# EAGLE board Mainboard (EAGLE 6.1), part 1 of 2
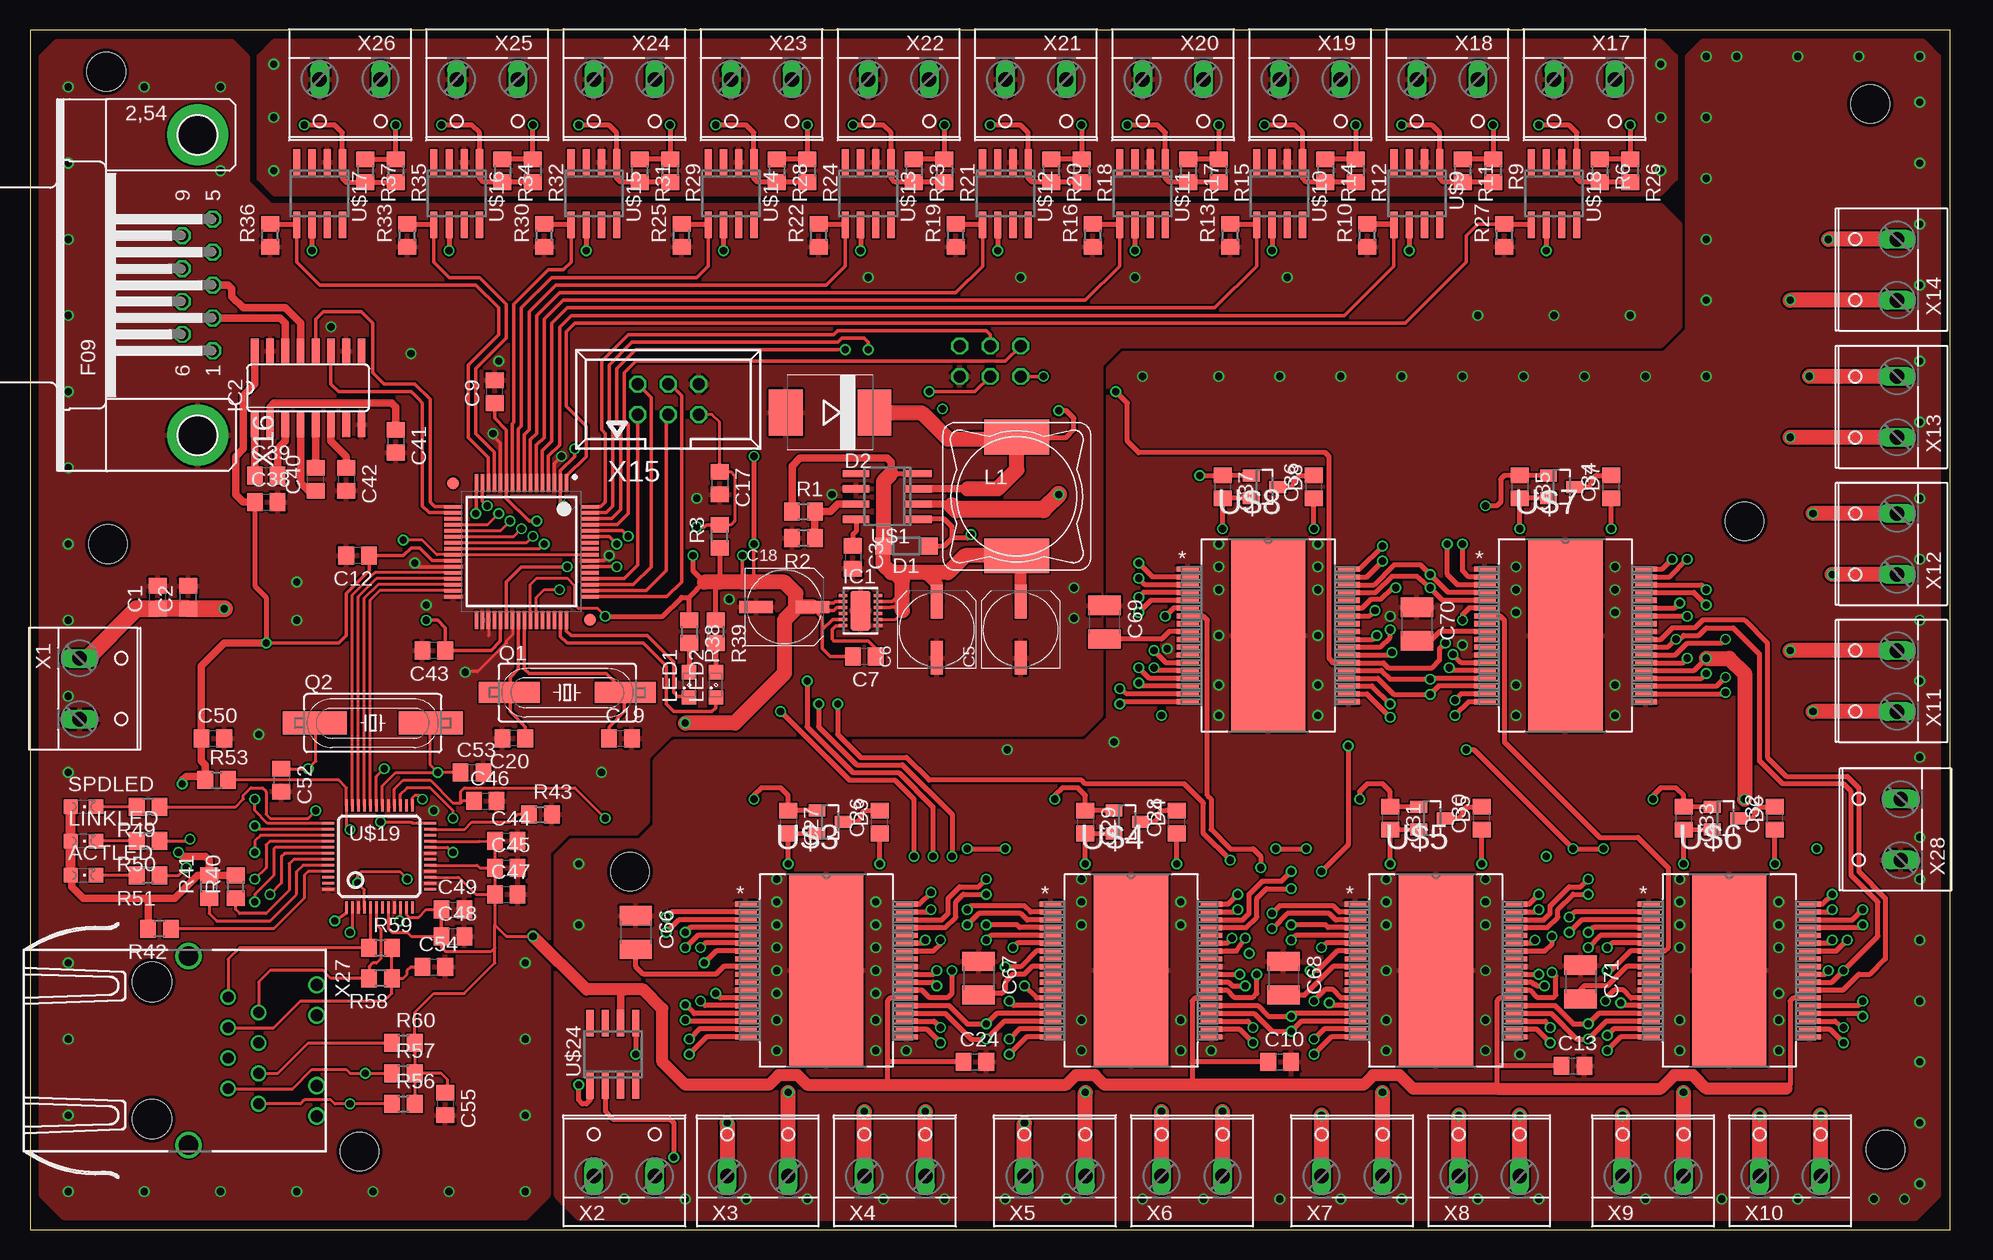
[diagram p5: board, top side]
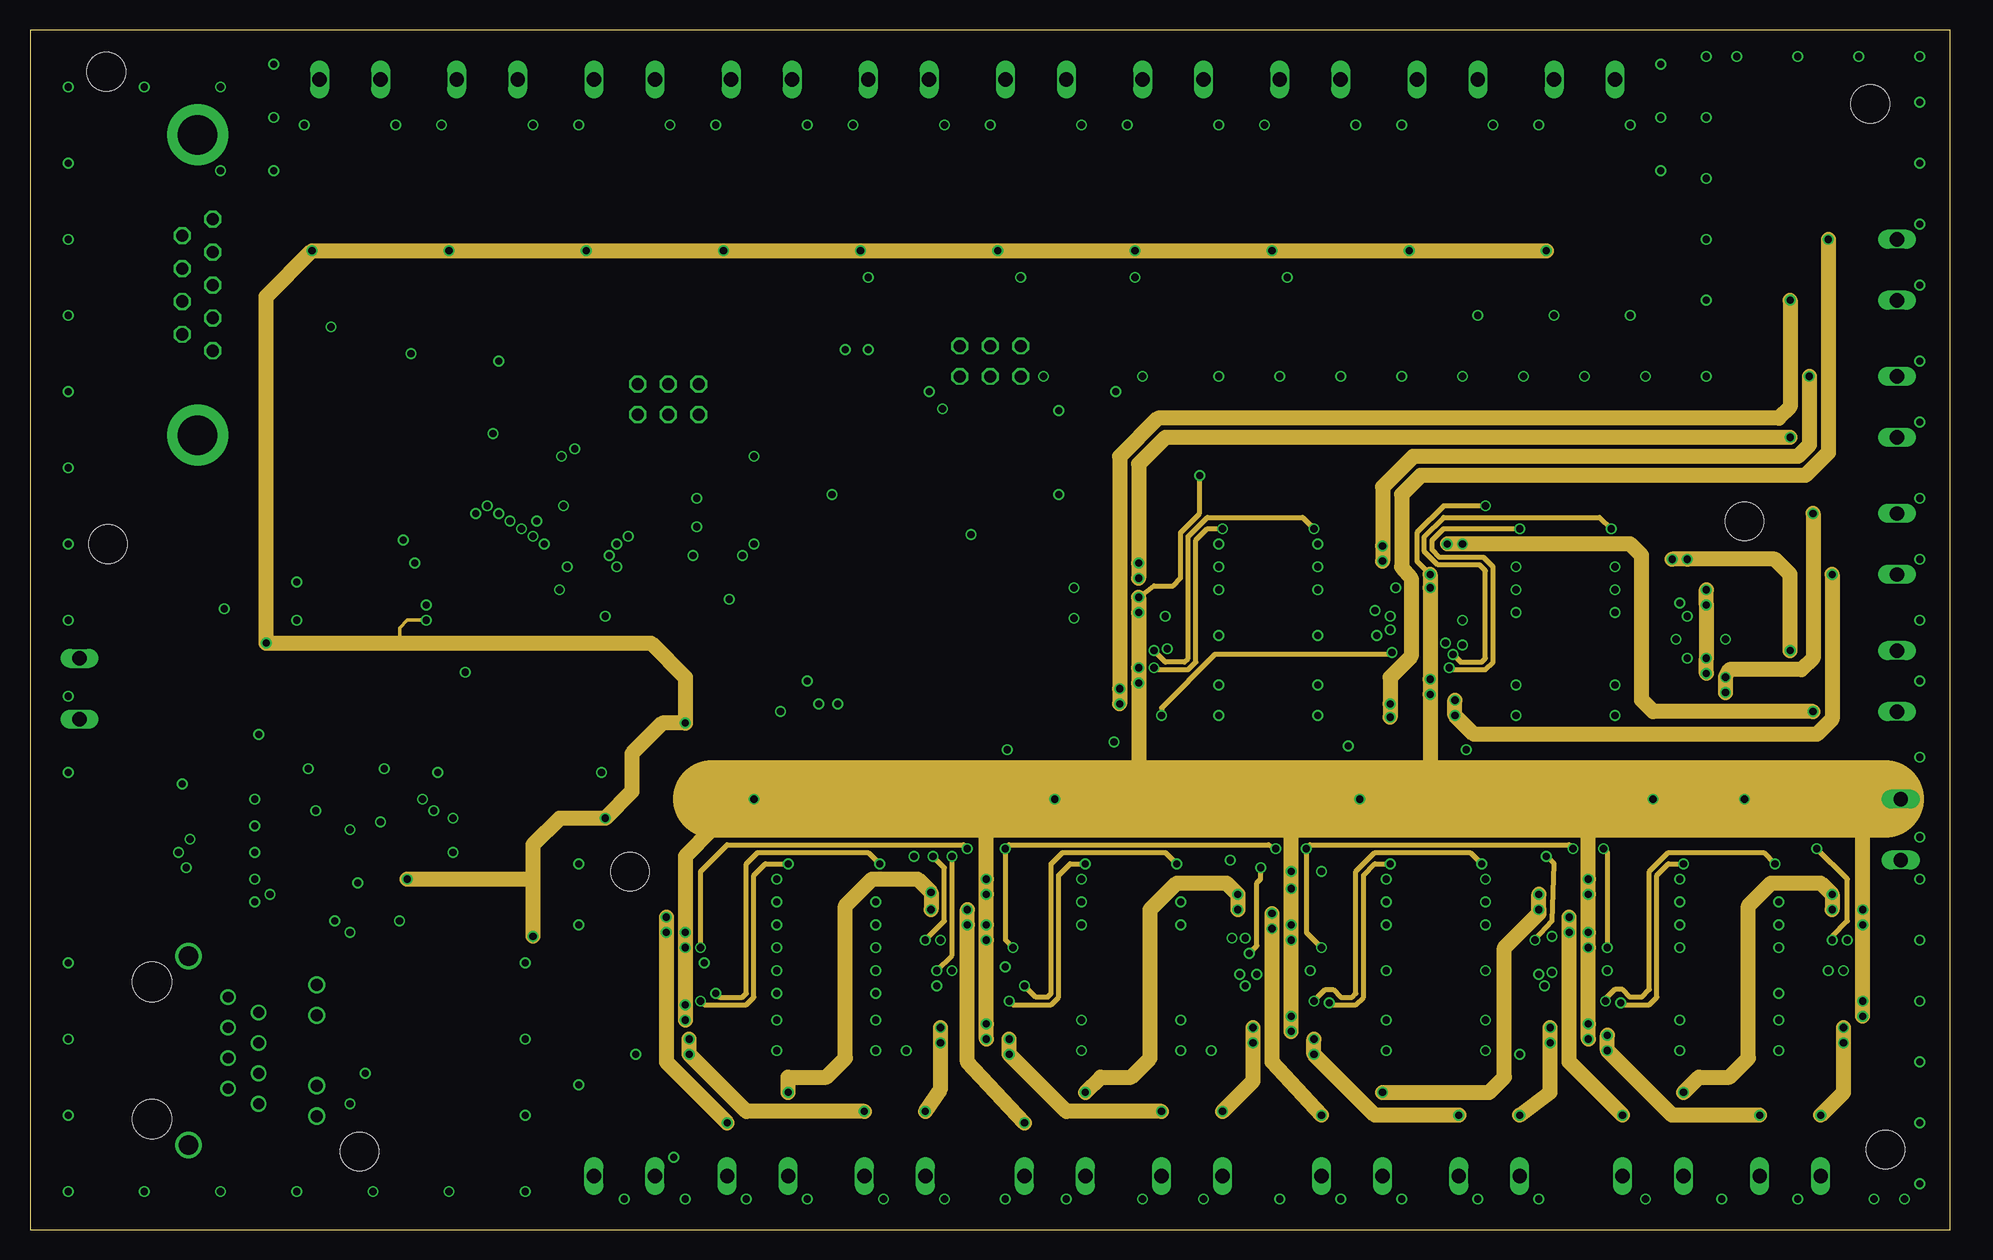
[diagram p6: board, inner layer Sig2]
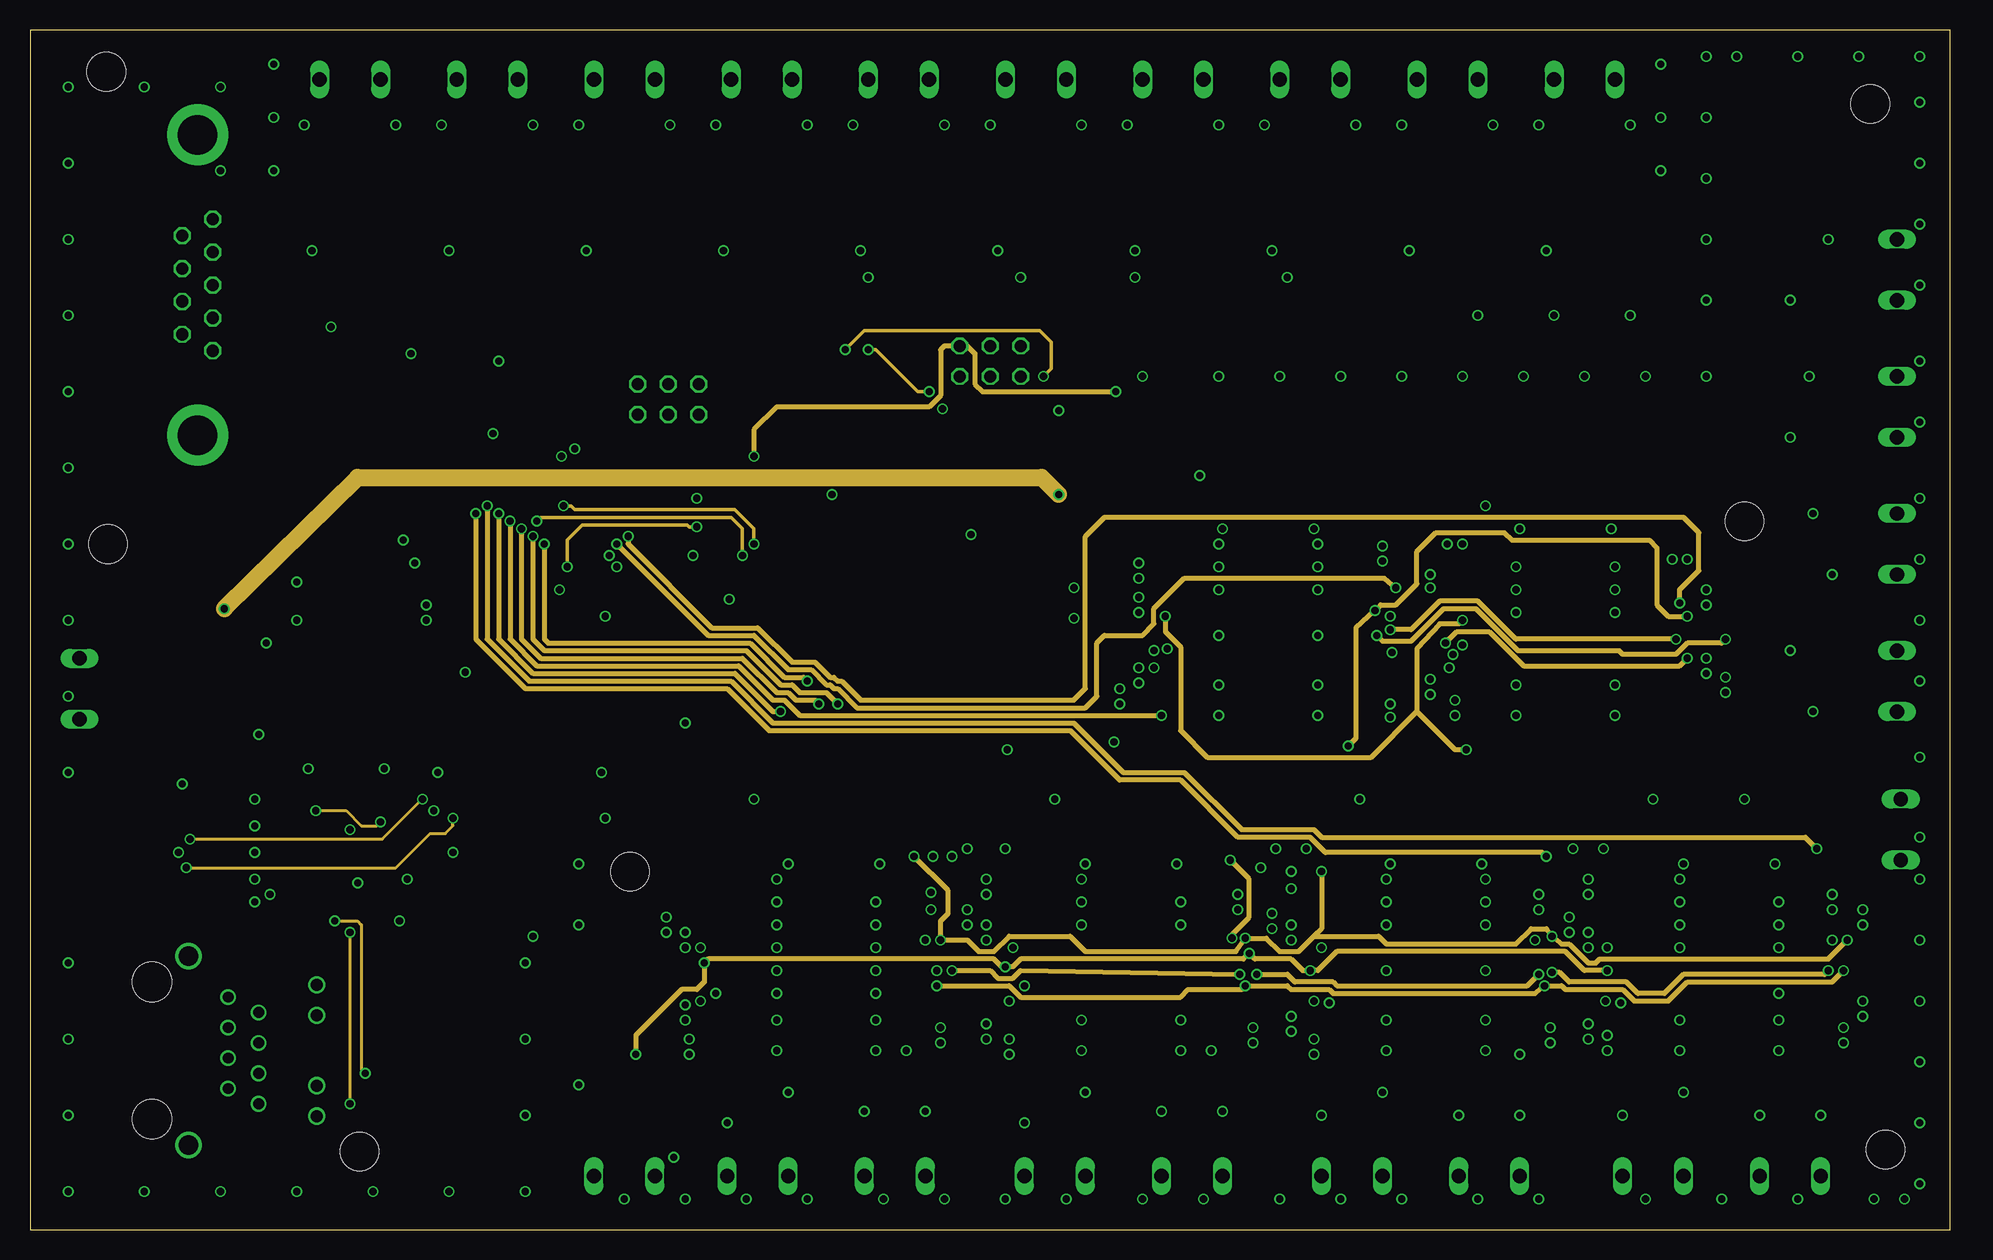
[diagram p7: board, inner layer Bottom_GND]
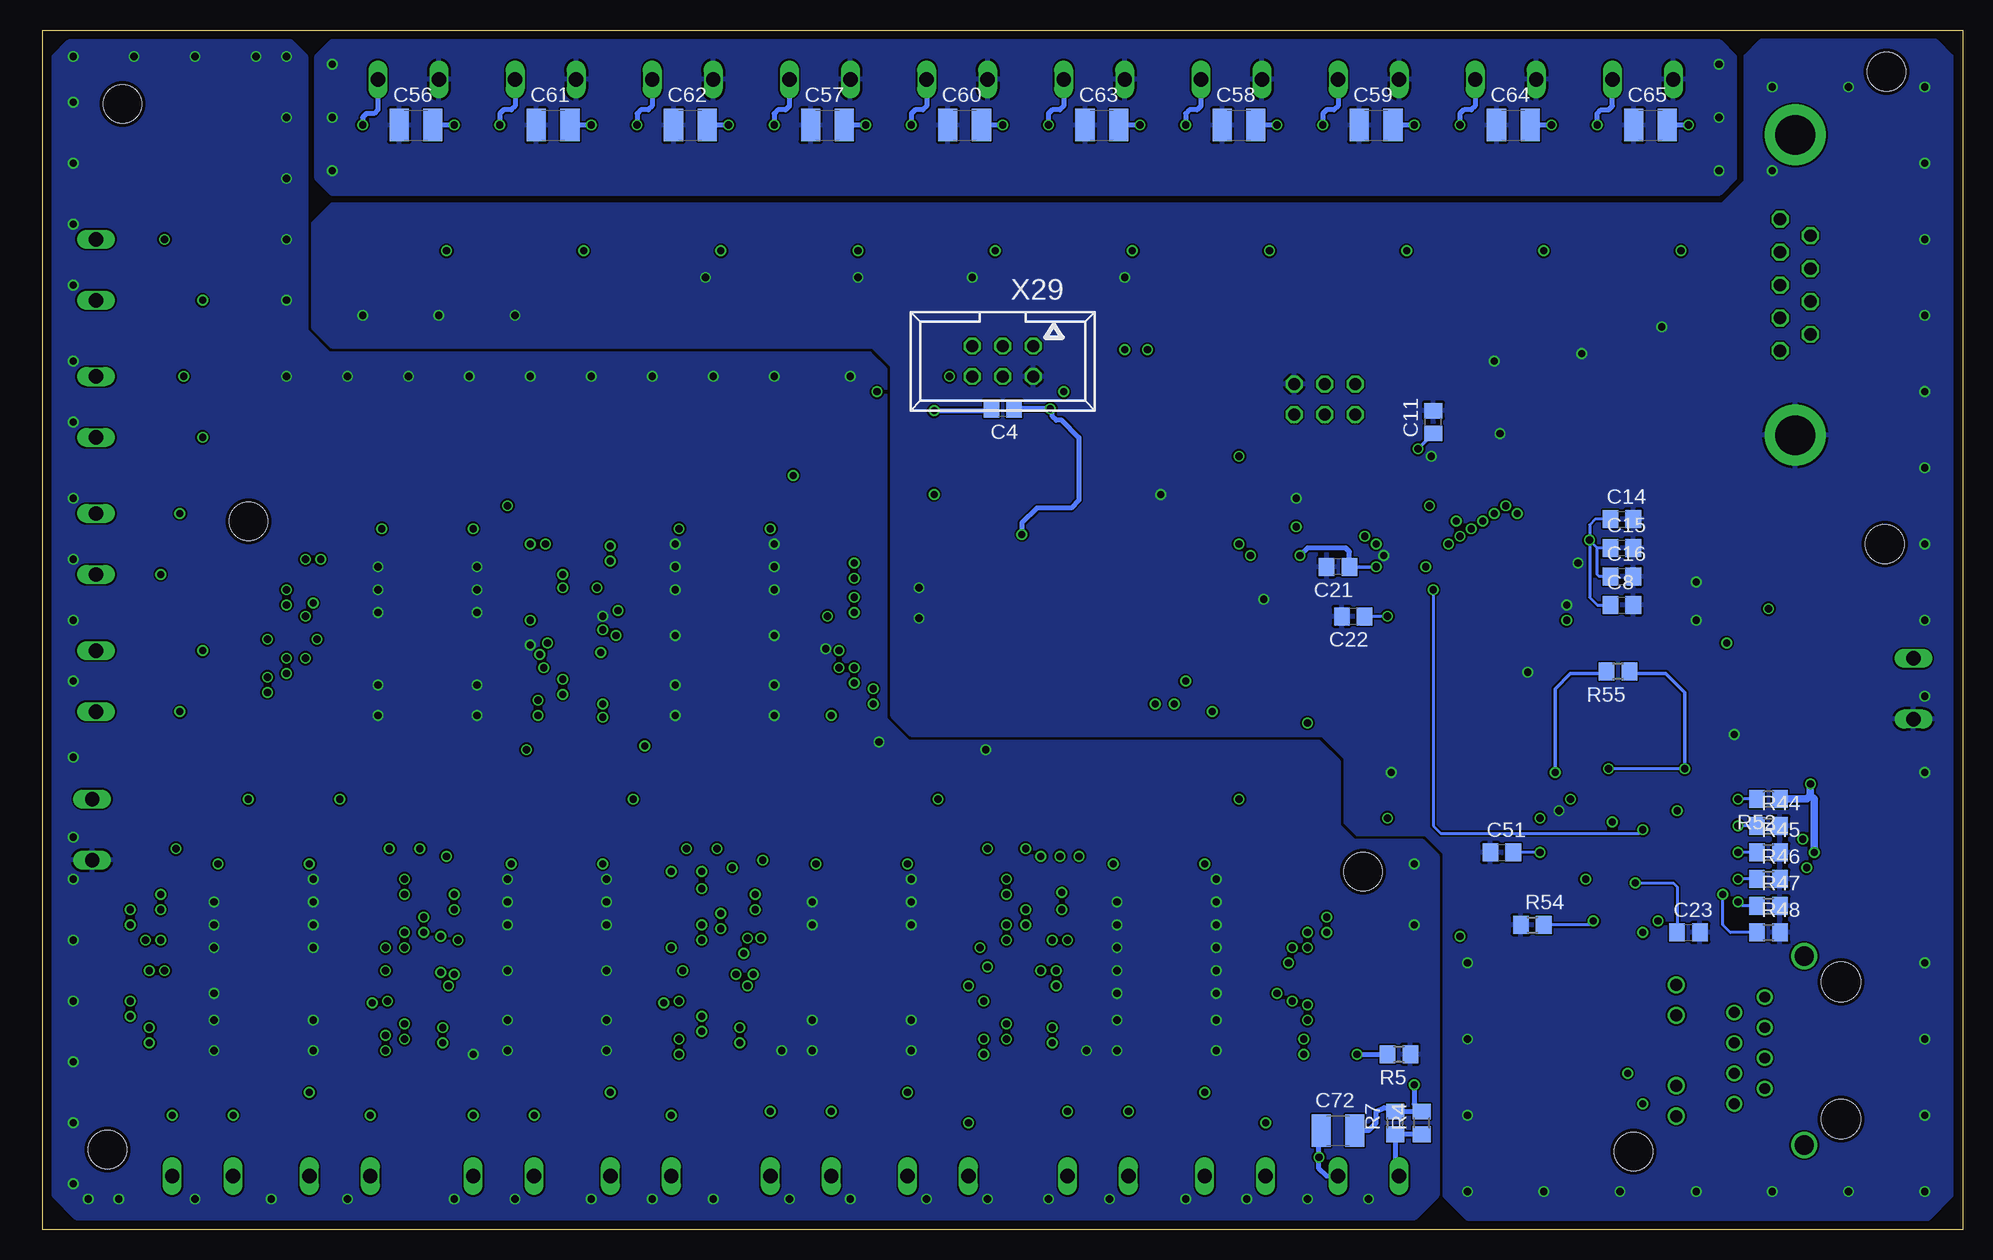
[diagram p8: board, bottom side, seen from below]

Size 160 x 100 mm. Coordinates in mm from the lower left corner, seen from the top.
Outline: 0,0 160,0 160,100 0,100 0,0
Copper layers (1+2*15+16): Sig1 0.035mm / dielectric 0.38mm / Sig2 0.035mm / dielectric 0.71mm / Bottom_GND 0.035mm / dielectric 0.38mm / Bottom 0.035mm
Design rules: minimum track width 0.15mm, minimum drill 0.3mm, track to track 0.15mm, track to pad 0.15mm, pad to pad 0.15mm, via to via 0.15mm, smd to smd 0.15mm, copper to edge 0.3mm, drill to drill 0.2mm, minimum pad ring 0.2mm, minimum via ring 0.15mm, stop-mask expansion 0.075mm, vias tented up to drill 0mil, thermal gap 0.2mm
Holes 3.2 mm at 142.88,59.05 154.62,6.67 27.46,6.51 50.01,29.84 6.35,96.52 6.51,57.15 153.35,93.82

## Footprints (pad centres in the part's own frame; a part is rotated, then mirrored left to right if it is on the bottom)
CHIPLED_0805 = smd 1.2 x 1.2: A 0,-1.05; C 0,1.05
C0805 = smd 1.3 x 1.5: 1 -0.95,0; 2 0.95,0
UD-6,3X7,7_NICHICON = smd 2.8 x 1: + 2.35,0; - -2.35,0
C1210 = smd 1.6 x 2.7: 1 -1.4,0; 2 1.4,0
SOD123 = smd 1.4 x 1.4: A 1.9,0; C -1.9,0
SMC = smd 2.8 x 3.8: A 3.7,0; C -3.7,0
SOT23 = smd 1 x 1.4: 1 -0.95,-1.1; 2 0.95,-1.1; 3 0,1.1
DFN12 = smd 0.25 x 0.7: 1 -1.25,-1.45; 2 -0.75,-1.45; 3 -0.25,-1.45; 4 0.25,-1.45; 5 0.75,-1.45; 6 1.25,-1.45; 7 1.25,1.45; 8 0.75,1.45; 9 0.25,1.45; 10 -0.25,1.45; 11 -0.75,1.45; 12 -1.25,1.45 | smd 3.3 x 1.7: EXP 0,0
SO16 = smd 0.66 x 2.032: 1 -4.445,-3.073; 2 -3.175,-3.073; 3 -1.905,-3.073; 4 -0.635,-3.073; 5 0.635,-3.073; 6 1.905,-3.073; 7 3.175,-3.073; 8 4.445,-3.073; 9 4.445,3.073; 10 3.175,3.073; 11 1.905,3.073; 12 0.635,3.073; 13 -0.635,3.073; 14 -1.905,3.073; 15 -3.175,3.073; 16 -4.445,3.073
PIS4720 = smd 5.4 x 2.9: P$1 0,4.95; P$2 0,-4.95
SML0805 = smd 1.2 x 1.2: A 1.05,0; C -1.05,0
SM49 = smd 5.08 x 1.778: 1 -4.826,0; 2 4.826,0
HC49UP = smd 5.334 x 1.93: 1 -4.826,0; 2 4.826,0
R0805 = smd 1.3 x 1.5: 1 -0.95,0; 2 0.95,0
SOIC8 = smd 0.6 x 2.2: 1 -1.905,-2.6; 2 -0.635,-2.6; 3 0.635,-2.6; 4 1.905,-2.6; 5 1.905,2.6; 6 0.635,2.6; 7 -0.635,2.6; 8 -1.905,2.6
QFP50P1200X1200X160-64N = smd 1.5 x 0.3: 1 -5.7,3.75; 2 -5.7,3.25; 3 -5.7,2.75; 4 -5.7,2.25; 5 -5.7,1.75; 6 -5.7,1.25; 7 -5.7,0.75; 8 -5.7,0.25; 9 -5.7,-0.25; 10 -5.7,-0.75; 11 -5.7,-1.25; 12 -5.7,-1.75; 13 -5.7,-2.25; 14 -5.7,-2.75; 15 -5.7,-3.25; 16 -5.7,-3.75; 33 5.7,-3.75; 34 5.7,-3.25; 35 5.7,-2.75; 36 5.7,-2.25; 37 5.7,-1.75; 38 5.7,-1.25; 39 5.7,-0.75; 40 5.7,-0.25; 41 5.7,0.25; 42 5.7,0.75; 43 5.7,1.25; 44 5.7,1.75; 45 5.7,2.25; 46 5.7,2.75; 47 5.7,3.25; 48 5.7,3.75 | smd 0.3 x 1.5: 17 -3.75,-5.7; 18 -3.25,-5.7; 19 -2.75,-5.7; 20 -2.25,-5.7; 21 -1.75,-5.7; 22 -1.25,-5.7; 23 -0.75,-5.7; 24 -0.25,-5.7; 25 0.25,-5.7; 26 0.75,-5.7; 27 1.25,-5.7; 28 1.75,-5.7; 29 2.25,-5.7; 30 2.75,-5.7; 31 3.25,-5.7; 32 3.75,-5.7; 49 3.75,5.7; 50 3.25,5.7; 51 2.75,5.7; 52 2.25,5.7; 53 1.75,5.7; 54 1.25,5.7; 55 0.75,5.7; 56 0.25,5.7; 57 -0.25,5.7; 58 -0.75,5.7; 59 -1.25,5.7; 60 -1.75,5.7; 61 -2.25,5.7; 62 -2.75,5.7; 63 -3.25,5.7; 64 -3.75,5.7 | smd 1 x 1: 65 -5.7,-5.7; 66 5.7,5.7
SOP65P1400X360-37N = smd 1.803 x 0.432: 1 -6.706,5.537; 2 -6.706,4.877; 3 -6.706,4.216; 4 -6.706,3.581; 5 -6.706,2.921; 6 -6.706,2.286; 7 -6.706,1.626; 8 -6.706,0.965; 9 -6.706,0.33; 10 -6.706,-0.33; 11 -6.706,-0.965; 12 -6.706,-1.626; 13 -6.706,-2.286; 14 -6.706,-2.921; 15 -6.706,-3.581; 16 -6.706,-4.216; 17 -6.706,-4.877; 18 -6.706,-5.537; 19 6.706,-5.537; 20 6.706,-4.877; 21 6.706,-4.216; 22 6.706,-3.581; 23 6.706,-2.921; 24 6.706,-2.286; 25 6.706,-1.626; 26 6.706,-0.965; 27 6.706,-0.33; 28 6.706,0.33; 29 6.706,0.965; 30 6.706,1.626; 31 6.706,2.286; 32 6.706,2.921; 33 6.706,3.581; 34 6.706,4.216; 35 6.706,4.877; 36 6.706,5.537 | smd 6.198 x 16.002: 37 0,0
LQFP48 = smd 0.2 x 1: 1 -2.75,-4.25; 2 -2.25,-4.25; 3 -1.75,-4.25; 4 -1.25,-4.25; 5 -0.75,-4.25; 6 -0.25,-4.25; 7 0.25,-4.25; 8 0.75,-4.25; 9 1.25,-4.25; 10 1.75,-4.25; 11 2.25,-4.25; 12 2.75,-4.25; 25 2.75,4.25; 26 2.25,4.25; 27 1.75,4.25; 28 1.25,4.25; 29 0.75,4.25; 30 0.25,4.25; 31 -0.25,4.25; 32 -0.75,4.25; 33 -1.25,4.25; 34 -1.75,4.25; 35 -2.25,4.25; 36 -2.75,4.25 | smd 1 x 0.2: 13 4.25,-2.75; 14 4.25,-2.25; 15 4.25,-1.75; 16 4.25,-1.25; 17 4.25,-0.75; 18 4.25,-0.25; 19 4.25,0.25; 20 4.25,0.75; 21 4.25,1.25; 22 4.25,1.75; 23 4.25,2.25; 24 4.25,2.75; 37 -4.25,2.75; 38 -4.25,2.25; 39 -4.25,1.75; 40 -4.25,1.25; 41 -4.25,0.75; 42 -4.25,0.25; 43 -4.25,-0.25; 44 -4.25,-0.75; 45 -4.25,-1.25; 46 -4.25,-1.75; 47 -4.25,-2.25; 48 -4.25,-2.75
W237-132 = drill 1.194 long: 1 -2.54,-0.635; 2 2.54,-0.635
057-006-1 = drill 1 octagon: 1 -2.54,-1.27; 2 -2.54,1.27; 3 0,-1.27; 4 0,1.27; 5 2.54,-1.27; 6 2.54,1.27
F09HP = drill 1.016 octagon: 1 -5.486,-1.27; 2 -2.743,-1.27; 3 0,-1.27; 4 2.743,-1.27; 5 5.486,-1.27; 6 -4.115,1.27; 7 -1.372,1.27; 8 1.372,1.27; 9 4.115,1.27 | drill 3.302 pad 5.08: G1 -12.522,0; G2 12.522,0
J1 = drill 0.9 pad 1.3: 1 4.445,2.54; 2 3.175,0; 3 1.905,2.54; 4 0.635,0; 5 -0.635,2.54; 6 -1.905,0; 7 -3.175,2.54; 8 -4.445,0 | drill 1 pad 1.422: 9 5.465,7.37; 10 2.925,7.37; 11 -2.925,7.37; 12 -5.465,7.37 | drill 1.6 pad 2.184: M1 -7.875,-3.3; M2 7.875,-3.3 | hole 3.3: 5.715,-6.35; -5.715,-6.35

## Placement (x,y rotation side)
ACTLED  [CHIPLED_0805]  4.45,29.53 270 top
C1  4µ7  [C0805]  10.64,52.7 90 top
C2  4µ7  [C0805]  13.18,52.7 90 top
C3  3n3  [C0805]  68.58,56.04 270 top
C4  100n  [C0805]  80.01,68.42 180 bottom
C5  100µ  [UD-6,3X7,7_NICHICON]  82.55,50.01 90 top
C6  100µ  [UD-6,3X7,7_NICHICON]  75.56,50.01 90 top
C7  10n  [C0805]  69.53,47.78 180 top
C8  1µ  [C0805]  28.42,52.07 0 bottom
C9  100n  [C0805]  38.73,69.85 90 top
C10  100n  [C0805]  104.14,13.97 0 top
C11  100n  [C0805]  44.13,67.31 90 bottom
C12  100n  [C0805]  27.3,56.2 180 top
C13  100n  [C0805]  128.59,13.65 0 top
C14  100n  [C0805]  28.42,59.21 0 bottom
C15  100n  [C0805]  28.42,56.83 0 bottom
C16  2µ2  [C0805]  28.42,54.45 0 bottom
C17  1n  [C0805]  57.47,62.23 270 top
C18  4µ7  [UD-6,3X7,7_NICHICON]  62.87,51.91 0 top
C19  10p  [C0805]  49.21,40.96 0 top
C20  10p  [C0805]  40.32,40.96 180 top
C21  10µ  [C0805]  52.07,55.24 180 bottom
C22  10µ  [C0805]  50.8,51.12 180 bottom
C23  47µ  [C0805]  22.86,24.77 0 bottom
C24  47µ  [C0805]  78.74,13.97 0 top
C26  10n  [C0805]  70.8,33.97 90 top
C27  220n  [C0805]  63.18,33.97 270 top
C28  10n  [C0805]  95.57,33.97 90 top
C29  220n  [C0805]  87.95,33.97 270 top
C30  10n  [C0805]  120.97,34.29 90 top
C31  220n  [C0805]  113.35,34.29 270 top
C32  10n  [C0805]  145.41,34.29 90 top
C33  220n  [C0805]  137.79,34.29 270 top
C34  10n  [C0805]  131.76,61.91 90 top
C35  220n  [C0805]  124.14,61.91 270 top
C36  10n  [C0805]  107,61.91 90 top
C37  220n  [C0805]  99.38,61.91 270 top
C38  100n  [C0805]  19.68,60.64 0 top
C39  100n  [C0805]  19.68,62.87 0 top
C40  100n  [C0805]  23.81,62.55 90 top
C41  100n  [C0805]  30.48,65.72 270 top
C42  100n  [C0805]  26.35,62.55 270 top
C43  100n  [C0805]  33.66,48.26 180 top
C44  100n  [C0805]  39.69,32.38 0 top
C45  100n  [C0805]  39.69,30.16 0 top
C46  100n  [C0805]  37.94,35.72 0 top
C47  100n  [C0805]  39.69,27.94 0 top
C48  100n  [C0805]  35.24,24.45 0 top
C49  100n  [C0805]  35.24,26.67 0 top
C50  100n  [C0805]  15.24,40.96 0 top
C51  4µ7  [C0805]  38.42,31.43 0 bottom
C52  18p  [C0805]  20.95,37.47 270 top
C53  18p  [C0805]  36.83,38.1 0 top
C54  100n  [C0805]  33.66,21.91 0 top
C55  10n  [C0805]  34.61,10.48 270 top
C56  [C1210]  128.91,92.08 0 bottom
C57  [C1210]  94.61,92.08 0 bottom
C58  [C1210]  60.33,92.08 0 bottom
C59  [C1210]  48.9,92.08 0 bottom
C60  [C1210]  83.19,92.08 0 bottom
C61  [C1210]  117.47,92.08 0 bottom
C62  [C1210]  106.05,92.08 0 bottom
C63  [C1210]  71.75,92.08 0 bottom
C64  [C1210]  37.47,92.08 0 bottom
C65  [C1210]  26.04,92.08 0 bottom
C66  [C1210]  50.48,24.77 270 top
C67  [C1210]  79.06,20.95 270 top
C68  [C1210]  104.46,20.95 270 top
C69  [C1210]  89.53,50.64 270 top
C70  [C1210]  115.57,50.48 270 top
C71  [C1210]  129.22,20.64 270 top
C72  [C1210]  52.07,8.26 0 bottom
D1  1N4148  [SOD123]  73.03,56.99 180 top
D2  MBRS340T3  [SMC]  66.67,68.1 180 top
D3  HSMS-2802-TR1G  [SOT23]  66.67,33.97 270 top
D4  HSMS-2802-TR1G  [SOT23]  91.44,33.97 270 top
D5  HSMS-2802-TR1G  [SOT23]  116.84,34.29 270 top
D6  HSMS-2802-TR1G  [SOT23]  141.29,34.29 270 top
D7  HSMS-2802-TR1G  [SOT23]  127.64,61.91 270 top
D8  HSMS-2802-TR1G  [SOT23]  102.87,61.91 270 top
IC1  LT1763CDE-3.3  [DFN12]  69.22,51.59 270 top
IC2  MAX3232CSE  [SO16]  23.18,70.17 0 top
L1  5µ  [PIS4720]  82.23,61.12 0 top
LED1  [SML0805]  54.93,45.4 90 top
LED2  [SML0805]  57.15,45.4 90 top
LINKLED  [CHIPLED_0805]  4.45,32.38 270 top
Q1  16M  [SM49]  44.77,44.77 0 top
Q2  25Mhz (1842313RL)  [HC49UP]  28.57,42.23 0 top
R1  5k6  [R0805]  64.45,59.85 0 top
R2  5k6  [R0805]  64.45,57.63 180 top
R3  [R0805]  57.47,57.78 90 top
R4  8k2  [R0805]  45.09,8.89 90 bottom
R5  100k  [R0805]  46.99,14.61 180 bottom
R6  8k2  [R0805]  130.81,88.27 270 top
R7  8k2  [R0805]  47.31,8.89 90 bottom
R9  8k2  [R0805]  121.92,88.27 270 top
R10  100k  [R0805]  111.44,82.87 90 top
R11  8k2  [R0805]  119.38,88.27 270 top
R12  8k2  [R0805]  110.49,88.27 270 top
R13  100k  [R0805]  100.01,82.87 90 top
R14  8k2  [R0805]  107.95,88.27 270 top
R15  8k2  [R0805]  99.06,88.27 270 top
R16  100k  [R0805]  88.58,82.87 90 top
R17  8k2  [R0805]  96.52,88.27 270 top
R18  8k2  [R0805]  87.63,88.27 270 top
R19  100k  [R0805]  77.15,82.87 90 top
R20  8k2  [R0805]  85.09,88.27 270 top
R21  8k2  [R0805]  76.2,88.27 270 top
R22  100k  [R0805]  65.72,82.87 90 top
R23  8k2  [R0805]  73.66,88.27 270 top
R24  8k2  [R0805]  64.77,88.27 270 top
R25  100k  [R0805]  54.29,82.87 90 top
R26  8k2  [R0805]  133.35,88.27 270 top
R27  100k  [R0805]  122.87,82.87 90 top
R28  8k2  [R0805]  62.23,88.27 270 top
R29  8k2  [R0805]  53.34,88.27 270 top
R30  100k  [R0805]  42.86,82.87 90 top
R31  8k2  [R0805]  50.8,88.27 270 top
R32  8k2  [R0805]  41.91,88.27 270 top
R33  100k  [R0805]  31.43,82.87 90 top
R34  8k2  [R0805]  39.37,88.27 270 top
R35  8k2  [R0805]  30.48,88.27 270 top
R36  100k  [R0805]  20,82.87 90 top
R37  8k2  [R0805]  27.94,88.27 270 top
R38  [R0805]  54.93,49.85 270 top
R39  [R0805]  57.15,49.85 270 top
R40  10k  [R0805]  17.14,28.57 90 top
R41  10k  [R0805]  14.92,28.57 90 top
R42  10k  [R0805]  10.79,25.08 180 top
R43  10k  [R0805]  42.55,34.61 0 top
R44  10k  [R0805]  16.19,33.66 0 bottom
R45  10k  [R0805]  16.19,31.43 0 bottom
R46  10k  [R0805]  16.19,29.21 0 bottom
R47  10k  [R0805]  16.19,26.99 0 bottom
R48  10k  [R0805]  16.19,24.77 0 bottom
R49  330R  [R0805]  9.84,35.24 180 top
R50  330R  [R0805]  9.84,32.38 180 top
R51  330R  [R0805]  9.84,29.53 180 top
R52  10k  [R0805]  16.19,35.88 180 bottom
R53  10k  [R0805]  15.56,37.47 0 top
R54  12k4 1%  [R0805]  35.88,25.4 0 bottom
R55  1M  [R0805]  28.73,46.51 180 bottom
R56  49R9  [R0805]  31.11,10.48 0 top
R57  49R9  [R0805]  31.11,13.02 0 top
R58  49R9  [R0805]  29.21,20.95 180 top
R59  49R9  [R0805]  29.21,23.5 0 top
R60  10R  [R0805]  31.11,15.56 0 top
SPDLED  [CHIPLED_0805]  4.45,35.24 270 top
U$1  LT1376  [SOIC8]  71.44,61.12 90 top
U$2  TM4C1233H6PM  [QFP50P1200X1200X160-64N]  40.96,56.52 270 top
U$3  L6470HPOWERSO36  [SOP65P1400X360-37N]  66.36,21.59 0 top
U$4  L6470HPOWERSO36  [SOP65P1400X360-37N]  91.76,21.59 0 top
U$5  L6470HPOWERSO36  [SOP65P1400X360-37N]  117.16,21.59 0 top
U$6  L6470HPOWERSO36  [SOP65P1400X360-37N]  141.6,21.59 0 top
U$7  L6470HPOWERSO36  [SOP65P1400X360-37N]  127.95,49.53 0 top
U$8  L6470HPOWERSO36  [SOP65P1400X360-37N]  103.19,49.53 0 top
U$9  IL217AT  [SOIC8]  115.57,86.36 180 top
U$10  IL217AT  [SOIC8]  104.14,86.36 180 top
U$11  IL217AT  [SOIC8]  92.71,86.36 180 top
U$12  IL217AT  [SOIC8]  81.28,86.36 180 top
U$13  IL217AT  [SOIC8]  69.85,86.36 180 top
U$14  IL217AT  [SOIC8]  58.42,86.36 180 top
U$15  IL217AT  [SOIC8]  46.99,86.36 180 top
U$16  IL217AT  [SOIC8]  35.56,86.36 180 top
U$17  IL217AT  [SOIC8]  24.13,86.36 180 top
U$18  IL217AT  [SOIC8]  127,86.36 180 top
U$19  W5500  [LQFP48]  29.11,31.12 0 top
U$24  IL217AT  [SOIC8]  48.58,14.61 0 top
X1  [W237-132]  4.76,45.09 270 top
X2  [W237-132]  49.53,5.08 0 top
X3  [W237-132]  60.64,5.08 0 top
X4  [W237-132]  72.07,5.08 0 top
X5  [W237-132]  85.41,5.08 0 top
X6  [W237-132]  96.84,5.08 0 top
X7  [W237-132]  110.17,5.08 0 top
X8  [W237-132]  121.6,5.08 0 top
X9  [W237-132]  135.25,5.08 0 top
X10  [W237-132]  146.69,5.08 0 top
X11  [W237-132]  154.94,45.72 90 top
X12  [W237-132]  154.94,57.15 90 top
X13  [W237-132]  154.94,68.58 90 top
X14  [W237-132]  154.94,80.01 90 top
X15  057-006-1  [057-006-1]  53.18,69.22 0 top
X16  [F09HP]  13.97,78.74 90 top
X17  [W237-132]  129.54,95.25 180 top
X18  [W237-132]  118.11,95.25 180 top
X19  [W237-132]  106.68,95.25 180 top
X20  [W237-132]  95.25,95.25 180 top
X21  [W237-132]  83.82,95.25 180 top
X22  [W237-132]  72.39,95.25 180 top
X23  [W237-132]  60.96,95.25 180 top
X24  [W237-132]  49.53,95.25 180 top
X25  [W237-132]  38.1,95.25 180 top
X26  [W237-132]  26.67,95.25 180 top
X27  J1006F21  [J1]  16.51,14.92 270 top
X28  [W237-132]  155.26,33.34 90 top
X29  057-006-1  [057-006-1]  80.01,72.39 180 bottom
